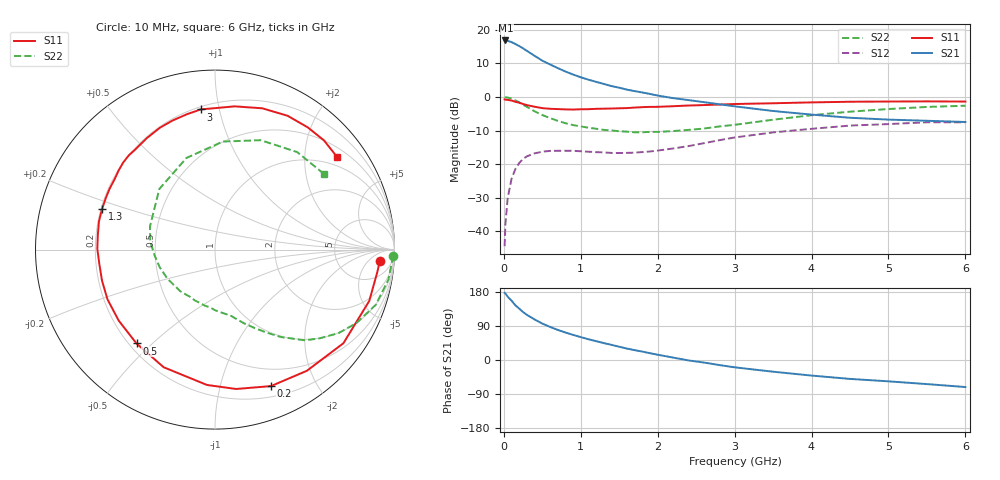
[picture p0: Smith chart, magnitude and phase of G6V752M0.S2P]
! SIEMENS Small Signal Semiconductors
! BFG193
! Si NPN RF Bipolar Junction Transistor in SOT223
! VCE = 0.75 V  IC = 2 mA
! Common Emitter S-Parameters:  August  1996
# GHz  S  MA  R  50
!  f  S11  S21  S12  S22
! GHz  MAG  ANG  MAG  ANG  MAG  ANG  MAG  ANG
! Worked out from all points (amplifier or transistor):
!   36 points, 10 MHz to 6 GHz, reference 50 ohm
!   highest |S21| = 16.8 dB at 20 MHz (marker M1)
!   |S21| within 3 dB of that: start of sweep to 292.8 MHz
!   unconditionally stable (mu >= 1): 1.339 GHz to 3.533 GHz; 5.554 GHz to end of sweep
!   at 250 MHz: K = 0.20, MSG = 16.5 dB, |S12| = -18.5 dB
!   at 1.4 GHz: K = 1.05, MAG = 8.6 dB, |S12| = -16.7 dB
!   at 6 GHz: K = 1.02, MAG = -0.8 dB, |S12| = -7.6 dB
!   S11 on the Smith chart (normalised r, x): 10 MHz: 15, -12; 200 MHz: 0.31, -1.45; 500 MHz: 0.23, -0.45; 1.3 GHz: 0.20, +0.17; 3 GHz: 0.22, +0.88; 6 GHz: 0.73, +2.80
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0.01  0.9208 -3.8  6.879 177.3  0.006 90.6  0.9942 -2.0
0.02  0.9133 -7.7  6.939 175.8  0.0125 87.2  0.9885 -3.9
0.05  0.9059 -18.4  6.842 167.0  0.0313 79.1  0.9805 -9.8
0.1  0.8854 -36.1  6.552 156.6  0.0603 70.3  0.9475 -18.9
0.15  0.8474 -52.8  6.14 144.4  0.0845 60.1  0.8883 -27.4
0.2  0.822 -67.7  5.731 135.6  0.1039 53.0  0.8315 -34.0
0.25  0.7854 -81.4  5.289 126.5  0.1194 45.9  0.7654 -40.2
0.3  0.7554 -93.4  4.852 119.1  0.1306 40.4  0.7123 -45.2
0.4  0.7151 -113.6  4.1 107.0  0.1447 31.5  0.6111 -52.9
0.5  0.6818 -129.9  3.471 96.1  0.1529 24.4  0.5381 -58.7
0.6  0.6666 -143.6  3.048 87.4  0.1575 19.6  0.4844 -63.7
0.7  0.66 -155.2  2.694 79.5  0.158 15.9  0.4421 -68.4
0.9  0.6494 -172.9  2.157 66.2  0.158 10.9  0.3812 -76.2
1.1  0.6579 172.8  1.808 54.8  0.1531 8.3  0.3485 -85.6
1.3  0.6687 160.2  1.562 44.7  0.1493 7.6  0.3231 -94.9
1.6  0.6827 145.2  1.284 30.1  0.1471 9.6  0.3046 -111.7
2.2  0.7282 121.4  0.961 6.4  0.1709 15.6  0.3105 -148.6
3  0.785 95.8  0.725 -19.3  0.2492 11.2  0.3844 160.5
3.5  0.8055 82.2  0.618 -30.9  0.2966 0.2  0.4585 132.6
4.5  0.8483 61.5  0.49 -49.9  0.3747 -20.7  0.6036 85.8
5.5  0.8595 45.1  0.442 -63.6  0.4195 -45.7  0.7105 49.9
6  0.854 37.2  0.424 -71.4  0.4191 -59.3  0.7402 34.5
